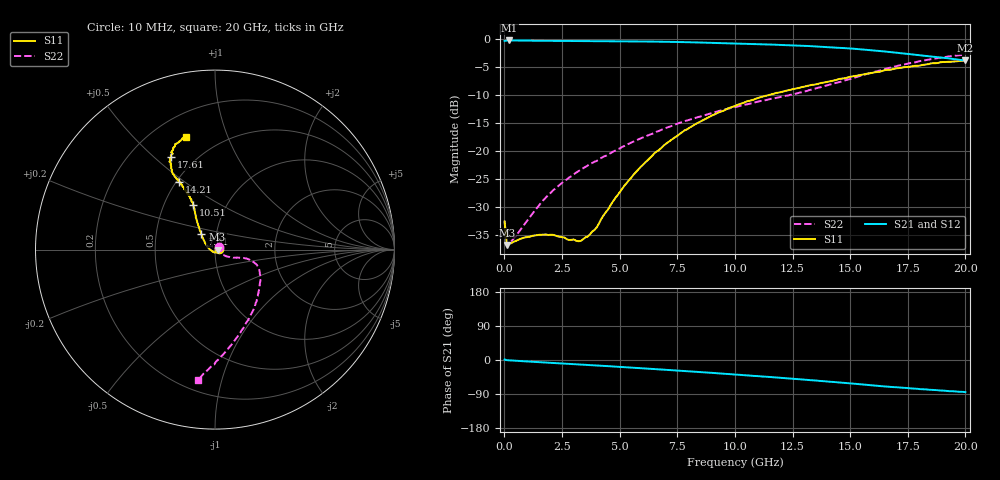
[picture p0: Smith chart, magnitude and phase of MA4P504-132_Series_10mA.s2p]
! AWR Design Environment (9226) Thu Aug 19 02:45:16 2021
! Document = '10mA'
! nPorts: 2, nXvals: 201
# GHz S DB R 50
!Freq DBS11 AngS11 DBS21 AngS21 DBS12 AngS12 DBS22 AngS22
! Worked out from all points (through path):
!   201 points, 10 MHz to 20 GHz, reference 50 ohm
!   highest |S21| = -0.17 dB at 210 MHz (marker M1); lowest = -3.8 dB at 20 GHz (marker M2)
!   group delay of S21, straight-line fit = 12 ps
!   lowest |S11| = -36.8 dB at 110 MHz (marker M3), VSWR 1.03, Z = 51.5 - j0.0391 ohm
!   |S11| at or under -10 dB: start of sweep to 11.42 GHz
!   |S22| runs from -37.0 to -2.7 dB; largest |S21 - S12| = 0.031
!   S11 on the Smith chart (normalised r, x): 10 MHz: 1.05, +0.01; 7.01 GHz: 0.84, +0.15; 10.51 GHz: 0.70, +0.38; 14.21 GHz: 0.52, +0.48; 17.61 GHz: 0.37, +0.57; 20 GHz: 0.33, +0.72
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0.01  -32.58 15.0  -0.26 1.2  -0.22 0.4  -32.62 30.9
0.11  -36.81 -1.5  -0.18 -0.4  -0.17 -0.5  -37.03 -2.5
0.21  -36.62 -1.5  -0.17 -0.8  -0.17 -0.9  -36.50 -1.7
0.91  -35.45 -16.1  -0.20 -3.6  -0.19 -3.5  -32.89 -16.2
1.81  -34.93 -43.5  -0.24 -6.8  -0.23 -6.6  -28.24 -28.0
3.21  -36.14 -111.7  -0.28 -11.6  -0.27 -11.3  -23.61 -31.3
3.41  -35.81 -124.8  -0.28 -12.4  -0.27 -12.0  -23.08 -30.8
4.01  -33.64 -162.3  -0.29 -14.6  -0.29 -14.1  -21.75 -28.8
4.81  -28.41 165.3  -0.31 -17.5  -0.31 -16.9  -19.91 -25.7
5.61  -24.19 147.8  -0.34 -20.5  -0.34 -19.8  -18.27 -21.7
6.71  -19.77 134.1  -0.39 -24.7  -0.39 -24.0  -16.37 -17.6
7.01  -18.68 131.7  -0.41 -25.9  -0.41 -25.1  -15.85 -17.0
8.31  -15.11 123.6  -0.52 -31.1  -0.52 -30.2  -14.02 -16.3
10.01  -11.90 116.6  -0.70 -38.4  -0.69 -36.9  -12.11 -20.0
10.51  -11.11 115.9  -0.76 -40.5  -0.74 -38.9  -11.64 -22.7
12.01  -9.41 115.6  -0.98 -47.1  -0.92 -45.5  -10.26 -34.5
13.41  -8.10 117.2  -1.22 -53.6  -1.13 -52.1  -8.87 -49.2
14.21  -7.41 118.1  -1.42 -57.7  -1.29 -56.1  -7.98 -57.8
16.71  -5.44 117.5  -2.24 -70.7  -2.13 -69.3  -5.09 -82.4
17.61  -4.85 115.3  -2.62 -74.8  -2.53 -74.0  -4.23 -88.4
19.01  -4.03 110.7  -3.25 -80.6  -3.27 -80.4  -3.22 -95.0
20  -3.76 104.5  -3.75 -84.8  -3.87 -84.2  -2.68 -97.3
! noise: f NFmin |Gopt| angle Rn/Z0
0.01  0  1  0  2e-20
2.21  0  1  0  2e-20
4.41  0  1  0  2e-20
6.61  0  1  0  2e-20
8.81  0  1  0  2e-20
11.11  0  1  0  2e-20
13.31  0  1  0  2e-20
15.51  0  1  0  2e-20
17.71  0  1  0  2e-20
20  0  1  0  2e-20
